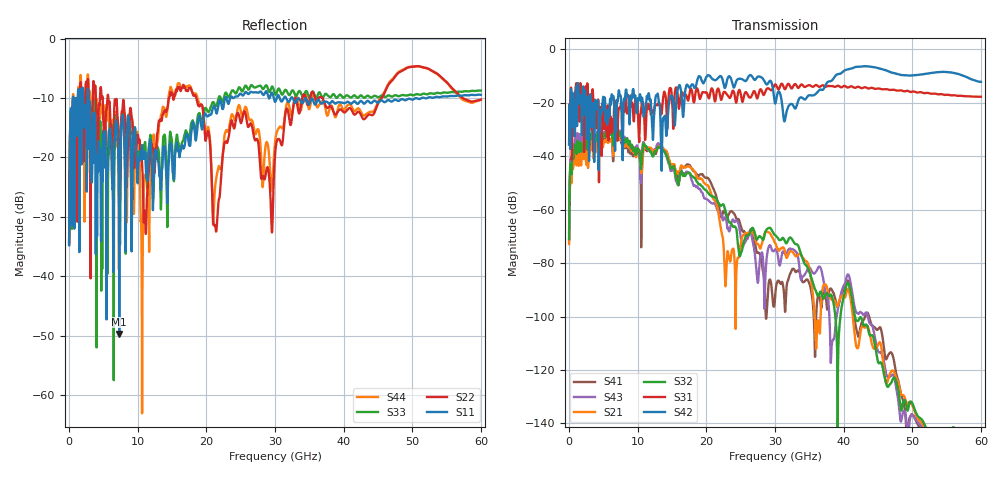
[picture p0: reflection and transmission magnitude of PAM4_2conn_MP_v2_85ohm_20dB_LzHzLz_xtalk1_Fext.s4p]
! Info: Touchstone file created by Circ.  Input file=FAB50GbE_2conn_Midplane_Examax_Topo2_v2_85ohm_20dB_LzHzLz.circ
# Hz S RI R 50
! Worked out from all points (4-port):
!   6000 points, 10 MHz to 60 GHz, reference 50 ohm
!   strongest paths, dB at 10 MHz, 15.01 GHz, 30.01 GHz, 45.01 GHz, 60 GHz:
!     S42: -35.6, -17.4, -20.2, -7.0, -12.1
!     S31: -35.5, -19.1, -13.1, -14.6, -17.7
!     S32: -71.1, -44.1, -69.5, -117.0, -150.7
!     S21: -72.8, -43.0, -72.4, -110.6, -146.2
!     S43: -70.8, -45.3, -74.9, -112.9, -152.9
!     S41: -68.6, -43.6, -93.1, -104.8, -154.4
!   lowest |S11| = -49.7 dB at 7.31 GHz (marker M1), VSWR 1.01, Z = 50 + j0.326 ohm
!   |S11| at or under -10 dB: 2.809 GHz to 22.74 GHz (19.93 GHz wide, 156 % of centre); 31.63 GHz to 32.33 GHz (707.8 MHz wide, 2.21 % of centre); 32.57 GHz to 51.37 GHz (18.8 GHz wide, 44.8 % of centre)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
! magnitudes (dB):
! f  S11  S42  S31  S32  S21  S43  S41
! 10 MHz  -34.8  -35.6  -35.5  -71.1  -72.8  -70.8  -68.6
! 1.07 GHz  -12.5  -14.3  -13.1  -38.3  -42.1  -35.2  -37.9
! 7.31 GHz  -49.7  -15.9  -21.8  -32.3  -33.7  -31.3  -33.5
! 13.61 GHz  -21.1  -29.1  -20.6  -37.6  -36.6  -37.6  -37.4
! 20.17 GHz  -13.1  -9.8  -17.0  -53.5  -50.8  -56.2  -48.0
! 22.87 GHz  -9.8  -13.3  -16.5  -61.0  -84.6  -63.8  -62.0
! 60 GHz  -9.5  -12.1  -17.7  -150.7  -146.2  -152.9  -154.4
